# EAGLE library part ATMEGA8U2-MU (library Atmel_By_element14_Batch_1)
Microcontroller with 8/16/32K Bytes of ISP Flash and USB Controller
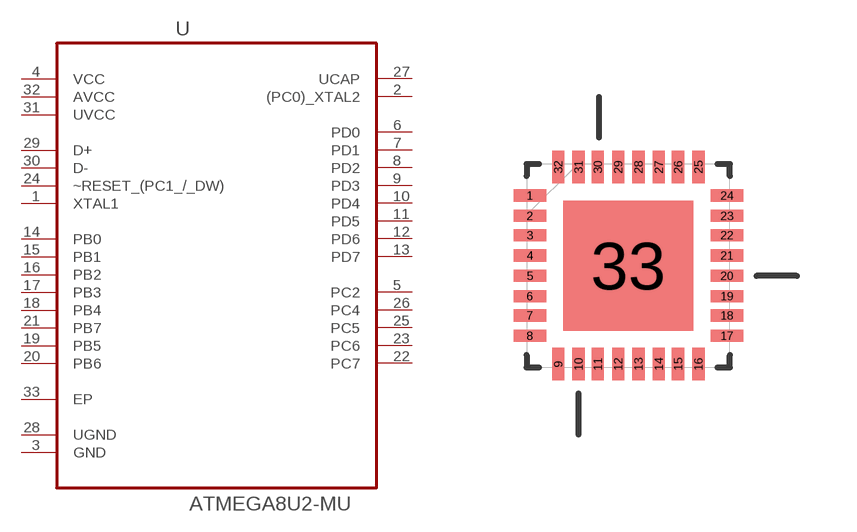
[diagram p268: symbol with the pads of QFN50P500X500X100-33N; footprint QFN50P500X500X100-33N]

Designator prefix U

## ATMEGA8U2-MU (MPN: ATMEGA8U2-MU; OC_FARNELL: 1748536; OC_NEWARK: 26R5642; PACKAGE: QFN-32; SUPPLIER: Atmel)  [QFN50P500X500X100-33N]
1  XTAL1  in
2  (PC0)_XTAL2
3  GND  pas
4  VCC  pwr
5  PC2
6  PD0
7  PD1
8  PD2
9  PD3
10  PD4
11  PD5
12  PD6
13  PD7
14  PB0
15  PB1
16  PB2
17  PB3
18  PB4
19  PB5
20  PB6
21  PB7
22  PC7
23  PC6
24  ~RESET_(PC1_/_DW)
25  PC5
26  PC4
27  UCAP  pwr
28  UGND  pas
29  D+  pas
30  D-  pas
31  UVCC  pwr
32  AVCC  pwr
33  EP  pas

## Footprint QFN50P500X500X100-33N (pad centres in mm)
smd 0.813 x 0.305: 1 -2.464,1.753; 2 -2.464,1.245; 3 -2.464,0.762; 4 -2.464,0.254; 5 -2.464,-0.254; 6 -2.464,-0.762; 7 -2.464,-1.245; 8 -2.464,-1.753; 17 2.464,-1.753; 18 2.464,-1.245; 19 2.464,-0.762; 20 2.464,-0.254; 21 2.464,0.254; 22 2.464,0.762; 23 2.464,1.245; 24 2.464,1.753
smd 0.305 x 0.813: 9 -1.753,-2.464; 10 -1.245,-2.464; 11 -0.762,-2.464; 12 -0.254,-2.464; 13 0.254,-2.464; 14 0.762,-2.464; 15 1.245,-2.464; 16 1.753,-2.464; 25 1.753,2.464; 26 1.245,2.464; 27 0.762,2.464; 28 0.254,2.464; 29 -0.254,2.464; 30 -0.762,2.464; 31 -1.245,2.464; 32 -1.753,2.464
smd 3.251 x 3.251: 33 0,0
